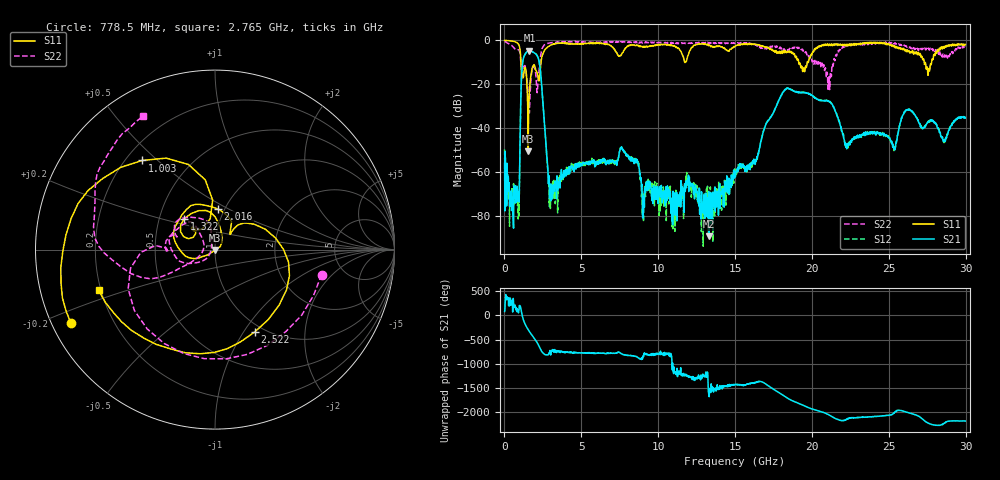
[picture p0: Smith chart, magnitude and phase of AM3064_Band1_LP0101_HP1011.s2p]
# Hz S DB R 50.0
!freq dBS11 angS11 dBS21 angS21 dBS12 angS12 dBS22 angS22
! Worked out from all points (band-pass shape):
!   1600 points, 10 MHz to 29.98 GHz, reference 50 ohm
!   highest |S21| = -4.69 dB at 1.622 GHz (marker M1); lowest = -89.5 dB at 13.32 GHz (marker M2)
!   |S21| within 3 dB of the highest: 1.254 GHz to 2.176 GHz (921.6 MHz wide, 53.7 % of centre)
!   lowest |S11| = -50.6 dB at 1.547 GHz (marker M3), VSWR 1.01, Z = 50.2 - j0.246 ohm
!   |S11| at or under -10 dB: 1.071 GHz to 2.378 GHz (1.307 GHz wide, 75.8 % of centre); 19.14 GHz to 19.7 GHz (559.4 MHz wide, 2.88 % of centre); 27.3 GHz to 27.78 GHz (479.6 MHz wide, 1.74 % of centre)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
!   |S22| runs from -33.2 to -0.4 dB; largest |S21 - S12| = 0.0087
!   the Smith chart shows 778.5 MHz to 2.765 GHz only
!   S11 on the Smith chart (normalised r, x): 778.5 MHz: 0.05, -0.24; 1.003 GHz: 0.27, +0.45; 1.322 GHz: 0.67, +0.25; 2.016 GHz: 0.93, +0.44; 2.522 GHz: 0.91, -1.12; 2.765 GHz: 0.19, -0.16
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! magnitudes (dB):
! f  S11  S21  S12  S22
! 10 MHz  0.0  -56.2  -49.8  -0.4
! 778.5 MHz  -0.9  -68.6  -72.8  -4.3
! 1.003 GHz  -3.9  -51.2  -50.8  -5.5
! 1.322 GHz  -12.3  -6.6  -6.5  -11.5
! 1.547 GHz  -50.6  -4.9  -4.7  -26.0
! 1.622 GHz  -23.3  -4.7  -4.7  -33.2
! 2.016 GHz  -12.9  -6.0  -6.0  -14.3
! 2.522 GHz  -5.9  -30.2  -30.1  -2.9
! 2.765 GHz  -3.3  -53.7  -53.5  -1.5
! 3.028 GHz  -2.0  -65.6  -72.5  -1.1
! 5.015 GHz  -1.4  -56.5  -56.6  -0.6
! 7.657 GHz  -5.8  -49.7  -49.5  -0.7
! 10 GHz  -2.0  -74.6  -70.2  -1.0
! 13.32 GHz  -2.1  -89.5  -72.9  -1.1
! 15 GHz  -2.6  -62.4  -58.8  -1.3
! 18.23 GHz  -5.5  -22.6  -22.6  -4.5
! 19.99 GHz  -6.6  -25.0  -25.1  -9.2
! 21.12 GHz  -1.7  -28.0  -27.7  -17.3
! 22.24 GHz  -2.1  -47.8  -48.4  -2.3
! 25 GHz  -1.5  -44.3  -44.0  -1.2
! 27.56 GHz  -15.1  -37.2  -37.2  -3.7
! 29.98 GHz  -1.8  -35.5  -35.2  -2.9
